TYPE Alarm :
STRUCT
	//PRESSURE_Warning:BOOL;
	PRESSURE:BOOL;
	
	//MFC1_Warning:BOOL;
	MFC1:BOOL;
	
	//MFC2_Warning:BOOL;
	MFC2:BOOL;
	
	//MFC3_Warning:BOOL;
	MFC3:BOOL;
	
	//MFC4_Warning:BOOL;
	MFC4:BOOL;
	
	//MFC5_Warning:BOOL;
	MFC5:BOOL;
	
	//MFC6_Warning:BOOL;
	MFC6:BOOL;
	
	//MFC7_Warning:BOOL;
	MFC7:BOOL;
	
	//MFC8_Warning:BOOL;
	MFC8:BOOL;
	
	//MFC9_Warning:BOOL;
	MFC9:BOOL;
	
	//WALL_TEMP_Warning:BOOL;
	WALL_TEMP:BOOL;
	
	//LID_TEMP_Warning:BOOL;
	LID_TEMP:BOOL;
	
	//STAGE_EDGE_TEMP_Warning:BOOL;
	STAGE_EDGE_TEMP:BOOL;
	
	//STAGE_CENTER_TEMP_Warning: BOOL;
	STAGE_CENTER_TEMP: BOOL;
	

	Gas1FlowPressureOutOfRange:BOOL;
	Gas2FlowPressureOutOfRange:BOOL;
	Gas3FlowPressureOutOfRange:BOOL;
	Gas4FlowPressureOutOfRange:BOOL;
	Gas5FlowPressureOutOfRange:BOOL;
	Gas6FlowPressureOutOfRange:BOOL;
	Gas7FlowPressureOutOfRange:BOOL;
	Gas8FlowPressureOutOfRange:BOOL;
	Gas9FlowPressureOutOfRange:BOOL;	
	
	
	TurboN2PurgePressureOutOfRange:BOOL;
	PrepareTransferTimerout:BOOL;
	TransferWaferTimeout:BOOL;
	OpenGasValveTimeout:BOOL;
	CloseGasValveTimeout:BOOL;
	OpenCloseSlitValveTimeout:BOOL;
	ATMCheckTimeout:BOOL;
	
	PLC:BOOL;	
	DRY_PUMP:BOOL;
	PENDULUM_VALVE:BOOL;
	TURBO_PUMP:BOOL;
	CHILLER1:BOOL;
	CHILLER2:BOOL;
	
	//PROCESS TOLERANCE
	TOLERANCE_PRESSURE:BOOL;
	TOLERANCE_MFC1:BOOL;
	TOLERANCE_MFC2:BOOL;
	TOLERANCE_MFC3:BOOL;
	TOLERANCE_MFC4:BOOL;
	TOLERANCE_MFC5:BOOL;
	TOLERANCE_MFC6:BOOL;
	TOLERANCE_MFC7:BOOL;
	TOLERANCE_MFC8:BOOL;
	TOLERANCE_MFC9:BOOL;
	TOLERANCE_WALL_TEMP:BOOL;
	TOLERANCE_LID_TEMP:BOOL;
	TOLERANCE_STAGE_EDGE_TEMP:BOOL;
	TOLERANCE_STAGE_CENTER_TEMP: BOOL;


	
END_STRUCT
END_TYPE
